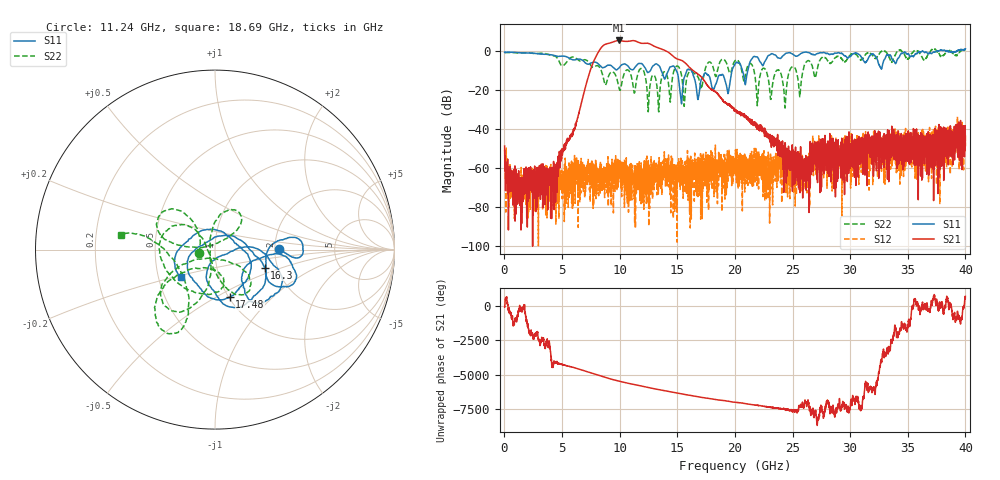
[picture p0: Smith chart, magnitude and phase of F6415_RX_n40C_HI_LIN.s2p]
!Keysight Technologies,N5245B,MY52451815,A.15.70.20
!Date: Wednesday, April 17, 2024 15:30:00
!Correction: S33(C  2-Port  )
!S43(C  2-Port  )
!S34(C  2-Port  )
!S44(C  2-Port  )
!S2P File: Measurements: S33, S43, S34, S44:
# Hz S  RI  R 50
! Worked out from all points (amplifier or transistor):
!   4000 points, 10 MHz to 40 GHz, reference 50 ohm
!   highest |S21| = 5.6 dB at 9.9 GHz (marker M1)
!   |S21| within 3 dB of that: 8.505 GHz to 13 GHz (4.498 GHz wide, 41.8 % of centre)
!   unconditionally stable (mu >= 1): start of sweep to 32.69 GHz; 33.07 GHz to 34.06 GHz; 34.49 GHz to 35.52 GHz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
!   at 6.67 GHz: K = 5233.34, MAG = -22.9 dB, |S12| = -61.3 dB
!   at 20.01 GHz: K = 8435.12, MAG = -27.6 dB, |S12| = -59.9 dB
!   at 40 GHz: K = 1134.85, MSG = -2.8 dB, |S12| = -42.8 dB
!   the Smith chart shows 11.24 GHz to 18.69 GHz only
!   S11 on the Smith chart (normalised r, x): 11.24 GHz: 2.12, +0.03; 16.3 GHz: 1.71, -0.37; 17.48 GHz: 1.01, -0.58; 18.69 GHz: 0.65, -0.21
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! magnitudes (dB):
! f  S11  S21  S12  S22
! 10 MHz  -0.4  -48.6  -50.6  -0.6
! 1.39 GHz  -0.7  -65.4  -65.7  -0.8
! 4.16 GHz  -1.8  -67.9  -63.8  -2.1
! 6.68 GHz  -4.3  -26.4  -67.5  -4.8
! 8.16 GHz  -6.6  -0.2  -66.9  -7.6
! 9.9 GHz  -8.7  5.6  -56.4  -17.8
! 11.24 GHz  -8.9  5.5  -65.0  -21.1
! 11.89 GHz  -6.2  4.2  -63.4  -8.9
! 13.34 GHz  -7.0  1.8  -62.4  -27.2
! 15.33 GHz  -25.5  -4.6  -60.5  -11.3
! 16.3 GHz  -10.6  -9.5  -62.8  -10.6
! 16.79 GHz  -24.7  -11.7  -63.7  -13.1
! 17.48 GHz  -11.1  -16.4  -51.9  -7.9
! 18.69 GHz  -12.2  -23.2  -64.4  -5.5
! 19.4 GHz  -21.7  -27.4  -59.6  -8.5
! 20.01 GHz  -6.5  -30.5  -59.9  -4.7
! 24.34 GHz  -1.4  -52.0  -57.0  -28.9
! 24.91 GHz  -1.1  -54.7  -54.7  -8.1
! 25.62 GHz  -1.5  -60.8  -55.5  -23.1
! 26.67 GHz  -1.5  -57.2  -55.7  -6.9
! 33.34 GHz  -2.0  -50.9  -44.2  -2.5
! 40 GHz  1.3  -48.4  -42.8  0.7
